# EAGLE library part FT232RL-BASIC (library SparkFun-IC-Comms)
FT232RL USB UART This is the simplified version of the FT232RL unit. Only what you need, nothing you don't. FT232RL 4th Generation USB UART (USB <-> Serial) Controller. Datasheet SparkFun Products Component (COM-00650) SparkFun RedBot Mainboard (ROB-12097) SparkFun FTDI Basic Breakout - 5V (DEV-09716) SparkFun FTDI Basic Breakout - 3.3V (DEV-09873) Bus Pirate - v3.6a (TOL-12942) SparkFun USB to Serial Breakout - FT232RL (BOB-12731) SparkFun PicoBoard (WIG-11888) SparkFun RFID USB Reader (SEN-09963) LilyPad FTDI Basic Breakout - 5V (DEV-10275) SparkFun Stepoko (ROB-13899)
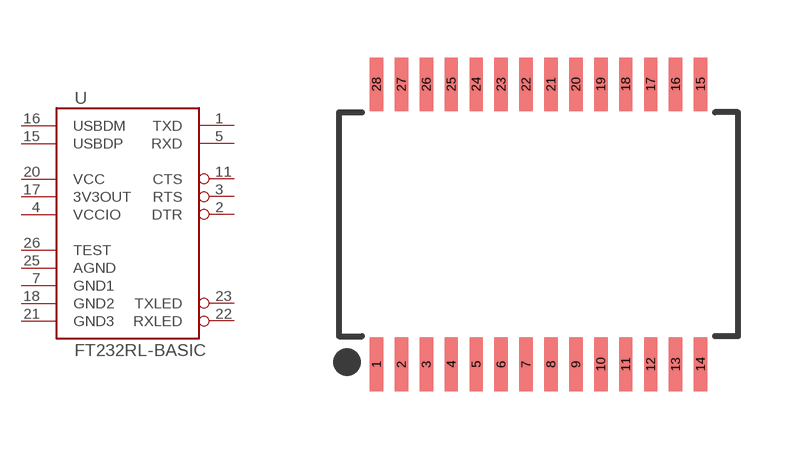
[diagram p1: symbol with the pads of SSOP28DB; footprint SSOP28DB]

Designator prefix U

## FT232RL-BASICSSOP (PROD_ID: IC-00870; VALUE: FT232RL)  [SSOP28DB]
1  TXD  out
2  DTR
3  RTS
4  VCCIO  pwr
5  RXD  in
7  GND1  pwr
11  CTS
15  USBDP
16  USBDM
17  3V3OUT  out
18  GND2  pwr
20  VCC  pwr
21  GND3  pwr
22  RXLED
23  TXLED
25  AGND  pwr
26  TEST  in

## Footprint SSOP28DB (pad centres in mm)
Small Shrink Outline Package - 28 DB Specifications: Pin count: 28 Example device(s): FT232RL
smd 0.348 x 1.397: 1 -4.225,-3.656; 2 -3.575,-3.656; 3 -2.925,-3.656; 4 -2.275,-3.656; 5 -1.625,-3.656; 6 -0.975,-3.656; 7 -0.325,-3.656; 8 0.325,-3.656; 9 0.975,-3.656; 10 1.625,-3.656; 11 2.275,-3.656; 12 2.925,-3.656; 13 3.575,-3.656; 14 4.225,-3.656; 15 4.225,3.656; 16 3.575,3.656; 17 2.925,3.656; 18 2.275,3.656; 19 1.625,3.656; 20 0.975,3.656; 21 0.325,3.656; 22 -0.325,3.656; 23 -0.975,3.656; 24 -1.625,3.656; 25 -2.275,3.656; 26 -2.925,3.656; 27 -3.575,3.656; 28 -4.225,3.656

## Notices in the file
Licensing: Creative Commons ShareAlike 4.0 International - https://creativecommons.org/licenses/by-sa/4.0
